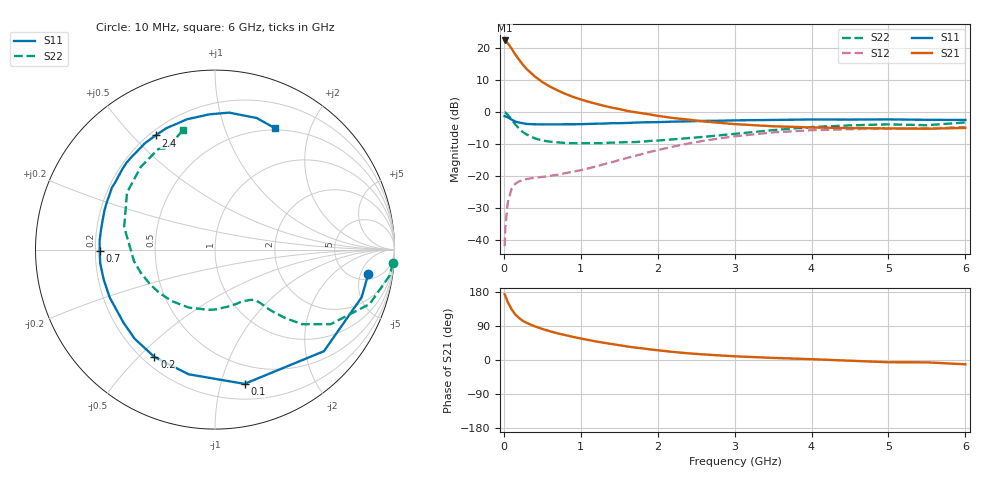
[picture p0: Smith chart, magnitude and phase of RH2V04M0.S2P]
! SIEMENS Small Signal Semiconductors
! BFR106
! Si NPN RF Bipolar Junction Transistor in SOT23
! VCE = 2 V  IC = 4 mA
! Common Emitter S-Parameters:  August  1996
# GHz  S  MA  R  50
!  f  S11  S21  S12  S22
! GHz  MAG  ANG  MAG  ANG  MAG  ANG  MAG  ANG
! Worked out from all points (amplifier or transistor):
!   36 points, 10 MHz to 6 GHz, reference 50 ohm
!   highest |S21| = 22.5 dB at 10 MHz (marker M1)
!   |S21| within 3 dB of that: start of sweep to 112.8 MHz
!   unconditionally stable (mu >= 1): 657.7 MHz to 2.183 GHz; 4.027 GHz to end of sweep
!   at 250 MHz: K = 0.45, MSG = 18.0 dB, |S12| = -21.3 dB
!   at 1.4 GHz: K = 1.19, MAG = 6.0 dB, |S12| = -15.7 dB
!   at 6 GHz: K = 1.03, MAG = -1.1 dB, |S12| = -4.7 dB
!   S11 on the Smith chart (normalised r, x): 10 MHz: 6.30, -6.83; 100 MHz: 0.33, -1.19; 200 MHz: 0.25, -0.56; 700 MHz: 0.22, -0.00; 2.4 GHz: 0.22, +0.58; 6 GHz: 0.48, +1.50
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0.01  0.8648 -9.1  13.31 173.7  0.0079 87.0  0.9936 -4.3
0.02  0.8593 -18.0  13.08 169.0  0.0159 80.1  0.9845 -8.4
0.05  0.83 -43.0  12.07 153.2  0.0377 67.8  0.9133 -19.4
0.1  0.7659 -77.6  9.988 134.1  0.0624 52.8  0.7669 -32.8
0.15  0.7101 -101.9  7.968 119.7  0.0754 42.7  0.6401 -40.5
0.2  0.687 -119.4  6.59 110.5  0.0822 37.7  0.5507 -44.1
0.25  0.6686 -132.0  5.502 102.9  0.0863 34.3  0.4837 -46.6
0.3  0.6524 -141.4  4.699 97.7  0.0895 33.3  0.4447 -48.0
0.4  0.6445 -155.6  3.656 89.0  0.0934 32.6  0.3893 -49.7
0.5  0.6422 -165.0  2.971 81.9  0.0962 33.9  0.3592 -51.6
0.6  0.6441 -173.1  2.517 75.8  0.1003 36.1  0.3444 -54.3
0.7  0.6427 -179.4  2.19 70.3  0.1042 38.8  0.3357 -57.7
0.9  0.6447 170.1  1.735 61.0  0.1167 44.8  0.3251 -64.4
1.1  0.6534 160.5  1.456 52.7  0.1313 50.2  0.3253 -73.5
1.6  0.6765 142.2  1.048 35.8  0.1908 57.2  0.3383 -97.8
2.2  0.7095 123.5  0.809 21.3  0.2878 54.3  0.3741 -129.8
2.4  0.7171 117.5  0.763 17.6  0.3226 51.5  0.3917 -141.5
3.5  0.7544 92.3  0.6 5.5  0.4804 30.8  0.5215 166.0
4.5  0.7642 77.8  0.562 -1.9  0.5396 12.2  0.6195 131.8
5  0.7691 72.4  0.556 -5.9  0.5509 4.9  0.6433 119.3
5.5  0.7579 67.1  0.55 -6.2  0.5591 1.5  0.6238 115.2
6  0.7539 63.6  0.565 -11.4  0.582 -6.0  0.6892 105.1
